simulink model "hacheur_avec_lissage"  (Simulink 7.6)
settings: Solver=ode23tb  StartTime=0.0  StopTime=20  RelTol=1e-3
StopFcn:
  | load Is_Ismoy_et_Ug.mat
  | plot(x(1,:),x(2,:),x(1,:),x(3,:),x(1,:),x(4,:))
  | grid
  | title('tension de sortie et sa valeur moyenne')
  | xlabel('temps')
libraries: powerlib x12, powerlib_extras x1

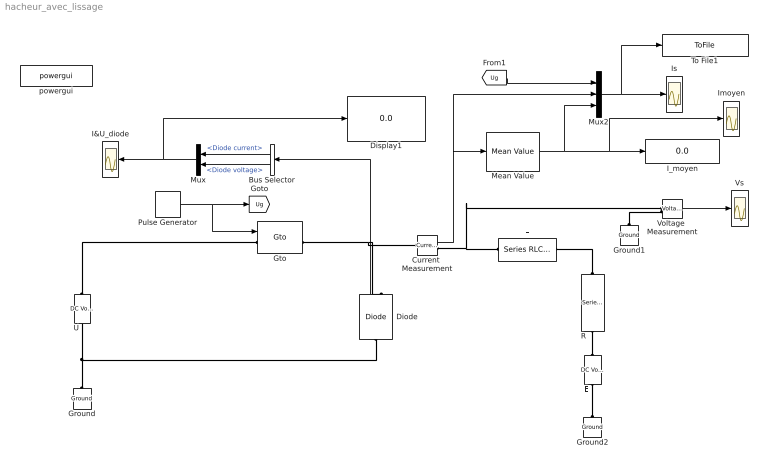
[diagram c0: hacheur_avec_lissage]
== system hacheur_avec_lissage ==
  Bus Selector : BusSelector  OutputSignals=Diode current,Diode voltage
  Current  Measurement : powerlib/Measurements/Current Measurement  DialogController=POWERSYS.PowerSysDialog  SystemSampleTime=-1  PhasorSimulation=off  OutputType=Complex  PSBequivalent=0
  Diode : powerlib/Power Electronics/Diode  DialogController=POWERSYS.PowerSysDialog  SystemSampleTime=-1  Ron=0.001  Lon=0  Vf=0.8  IC=0  UseSnubber=off  Rs=500  Cs=250e-9  Measurements=on
  Display1 : Display
  E : powerlib/Electrical Sources/DC Voltage Source  DialogController=POWERSYS.PowerSysDialog  SystemSampleTime=-1  Amplitude=6  Measurements=None
  Ground : powerlib/Elements/Ground  DialogController=POWERSYS.PowerSysDialog  PhysicalDomain=powersysdomain  SubClassName=unknown  LeftPortType=p1  RightPortType=p1  LConnTagsString=a
  Ground1 : powerlib/Elements/Ground  DialogController=POWERSYS.PowerSysDialog  PhysicalDomain=powersysdomain  SubClassName=unknown  LeftPortType=p1  RightPortType=p1  LConnTagsString=a
  Ground2 : powerlib/Elements/Ground  DialogController=POWERSYS.PowerSysDialog  PhysicalDomain=powersysdomain  SubClassName=unknown  LeftPortType=p1  RightPortType=p1  LConnTagsString=a
  Gto : powerlib/Power Electronics/Gto  DialogController=POWERSYS.PowerSysDialog  SystemSampleTime=-1  Ron=0.001  Lon=0  Vf=1  Tf=10e-6  Tt=20e-6  IC=0  Rs=1e5  Cs=inf  Measurements=on
  I&U_diode : Scope
  I_moyen : Display
  Imoyen : Scope
  Is : Scope
  L : powerlib/Elements/Series RLC Branch  DialogController=POWERSYS.PowerSysDialog  PhysicalDomain=powersysdomain  SubClassName=unknown  LeftPortType=p1  RightPortType=p1  LConnTagsString=__new0  RConnTagsString=__new0  BranchType=L  Resistance=100  Inductance=1  SetiL0=off  InitialCurrent=0  Capacitance=1e-6  Setx0=off  InitialVoltage=0  Measurements=None
  Mean Value : powerlib_extras/Measurements/Mean Value  DialogController=POWERSYS.PowerSysDialog  SystemSampleTime=-1  Period=10
  Mux : Mux  Inputs=2
  Mux2 : Mux  Inputs=3
  Pulse Generator : DiscretePulseGenerator  PulseType=Time based  Period=0.1  PulseWidth=60
  R : powerlib/Elements/Series RLC Branch  DialogController=POWERSYS.PowerSysDialog  PhysicalDomain=powersysdomain  SubClassName=unknown  LeftPortType=p1  RightPortType=p1  LConnTagsString=__new0  RConnTagsString=__new0  BranchType=R  Resistance=1  Inductance=1e-3  SetiL0=off  InitialCurrent=0  Capacitance=1e-6  Setx0=off  InitialVoltage=0  Measurements=None
  To File1 : ToFile  Filename=Is_Ismoy_et_Ug  MatrixName=x
  U : powerlib/Electrical Sources/DC Voltage Source  DialogController=POWERSYS.PowerSysDialog  SystemSampleTime=-1  Amplitude=15  Measurements=None
  Voltage  Measurement : powerlib/Measurements/Voltage Measurement  DialogController=POWERSYS.PowerSysDialog  SystemSampleTime=-1  PhasorSimulation=off  OutputType=Complex  PSBequivalent=0
  Vs : Scope
  powergui : powerlib/powergui  Priority=2  SystemSampleTime=-1  SimulationMode=Continuous  SampleTime=0  frequency=60  SPID=off  DisableSnubberDevices=off  DisableRonSwitches=off  DisableVfSwitches=off  SwTol=0  Interpol=off  frequencyindice=0  echomessages=off  HookPort=off  DisplayEquations=off  FunctionMessages=off  EnableUseOfTLC=off  x0status=blocks  RestoreLinks=warning  ResistiveCurrentMeasurement=off  Frange=logspace(0,3,50)  Ylog=off  Xlog=off  ShowGrid=off  save=off  variable=ZData  ZoomFFT=on  StartTime=0.0  cycles=1  DisplayStyle=off  fundamental=60  FreqAxis=off  MaxFrequency=1000  frequencyindicesteady=1  RmsSteady=1  display=off  Ts=0  methode=off
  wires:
  Pulse Generator/1 -> Gto/1, [Ug]
  Voltage  Measurement/1 -> Vs/1
  Current  Measurement/1 -> Mean Value/1, Mux2/2
  Mean Value/1 -> I_moyen/1, Imoyen/1, Mux2/3
  Diode/1 -> Bus Selector/1
  Bus Selector/1 -> Mux/1  "<Diode current>"
  Bus Selector/2 -> Mux/2  "<Diode voltage>"
  Mux/1 -> I&U_diode/1, Display1/1
  [Ug] -> Mux2/1
  Mux2/1 -> Is/1, To File1/1
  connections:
  Diode/LConn1 -- U/LConn1 -- Ground/LConn1
  U/RConn1 -- Gto/LConn1
  Gto/RConn1 -- Diode/RConn1 -- Current  Measurement/LConn1
  Ground1/LConn1 -- Voltage  Measurement/LConn2
  R/LConn1 -- L/LConn1
  R/RConn1 -- E/RConn1
  E/LConn1 -- Ground2/LConn1
  Current  Measurement/RConn1 -- L/RConn1 -- Voltage  Measurement/LConn1
